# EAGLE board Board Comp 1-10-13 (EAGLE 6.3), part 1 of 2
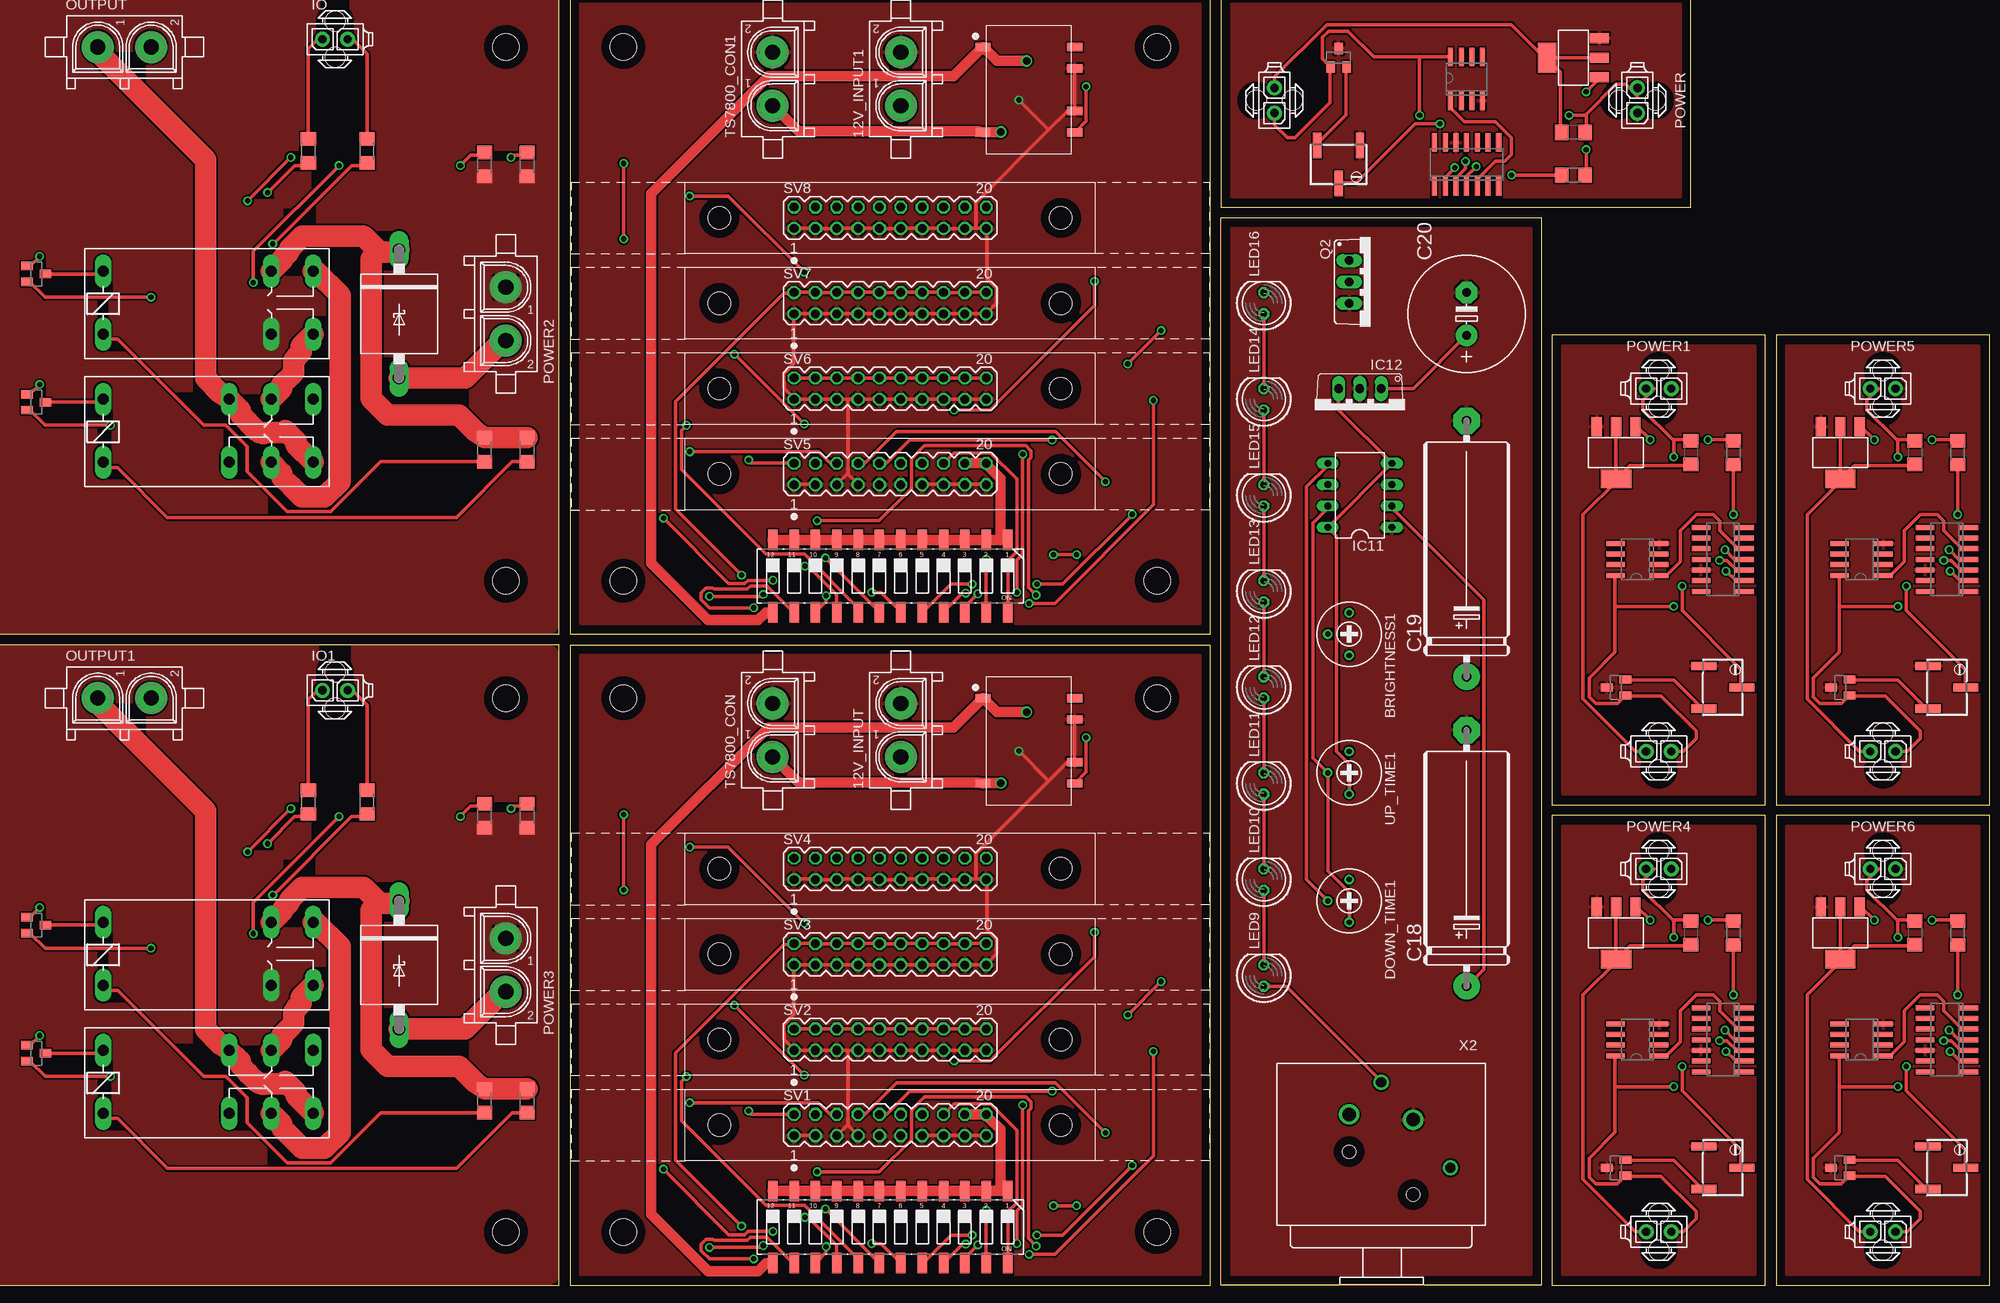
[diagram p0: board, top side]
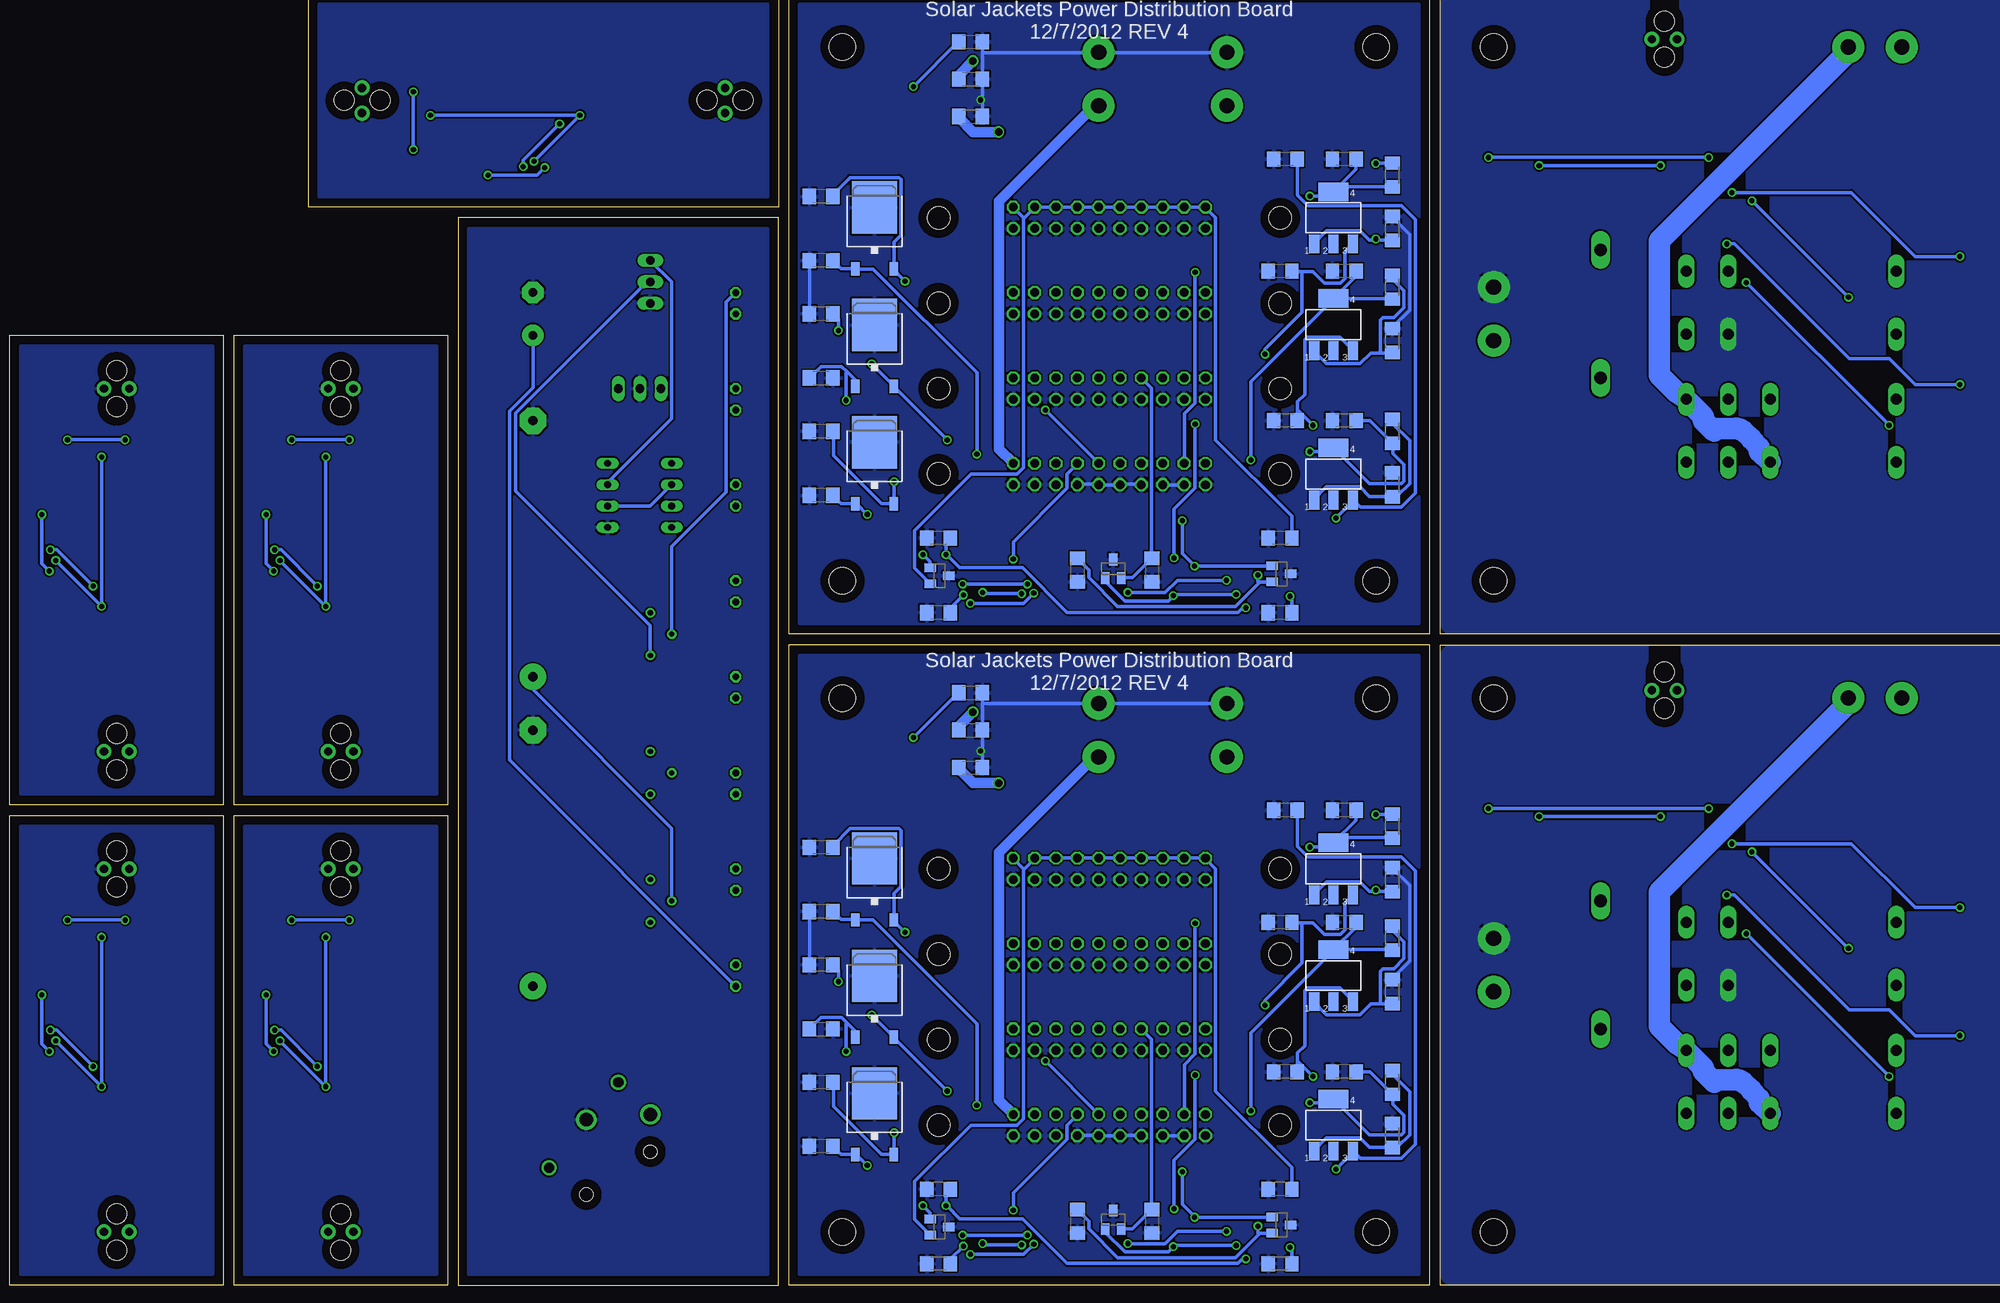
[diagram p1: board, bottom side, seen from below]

No outline drawn. Coordinates in mm, seen from the top.
Copper layers (1*16): Top 0.035mm / dielectric 1.5mm / Bottom 0.035mm
Design rules "default": minimum track width 10mil, minimum drill 24mil, track to track 8mil, track to pad 8mil, pad to pad 8mil, via to via 8mil, smd to smd 8mil, copper to edge 40mil, drill to drill 8mil, minimum pad ring 10mil, minimum via ring 8mil, stop-mask expansion 4mil, vias tented up to drill 0mil, thermal gap 10mil
Net classes: 1 power: width 1.27 mm, drill 0.889 mm
Holes 3.17 mm at 147.32,6.35 83.82,6.35 83.82,69.85 147.32,69.85 147.32,83.82 83.82,83.82 83.82,147.32 147.32,147.32 6.58,84 69.85,147.32 69.85,83.82 6.35,147.32 6.58,6.53 69.85,69.85 69.85,6.35 6.35,69.85
Milling: 40 lines

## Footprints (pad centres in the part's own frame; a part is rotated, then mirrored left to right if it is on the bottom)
SOT23 = smd 1 x 1.4: 1 -0.95,-1.1; 2 0.95,-1.1; 3 0,1.1
350759-4 = drill 1.8 pad 3.81: 1 -3.175,0; 2 3.175,0
C1206 = smd 1.6 x 1.8: 1 -1.4,0; 2 1.4,0
RTRIM3339P = drill 0.61: 1 -2.54,0; 2 0,-2.54; 3 2.54,0
E30-10 = drill 1.118 pad 3.15: + -15.24,0 | drill 1.118 pad 3.15 octagon: - 15.24,0
E5-13 = drill 1.016 pad 2.54: + -2.54,0 | drill 1.016 pad 2.54 octagon: - 2.54,0
P6T15 = drill 1.499 long: A 7.62,0; C -7.62,0
SO14 = smd 0.6 x 2.2: 1 -3.81,-2.6; 2 -2.54,-2.6; 3 -1.27,-2.6; 4 0,-2.6; 5 1.27,-2.6; 6 2.54,-2.6; 7 3.81,-2.6; 8 3.81,2.6; 9 2.54,2.6; 10 1.27,2.6; 11 0,2.6; 12 -1.27,2.6; 13 -2.54,2.6; 14 -3.81,2.6
SOT223 = smd 1.219 x 2.235: 1 -2.311,-3.099; 2 0,-3.099; 3 2.311,-3.099 | smd 3.6 x 2.2: 4 0,3.099
DIL08 = drill 0.813 long: 1 -3.81,-3.81; 2 -1.27,-3.81; 3 1.27,-3.81; 4 3.81,-3.81; 5 3.81,3.81; 6 1.27,3.81; 7 -1.27,3.81; 8 -3.81,3.81
TO220V = drill 1.016 long: 1 -2.54,-2.54; 2 0,-2.54; 3 2.54,-2.54
794681-2 = drill 1 pad 1.778: 1 0,-1.5; 2 0,1.5 | hole 2.4: 2.13,0; -2.17,0
G2R2 = drill 1.321 long: 1 -2.54,-3.683; 2 -2.54,3.81; O1 12.471,3.81; O2 12.471,-3.683; P1 17.45,3.81; P2 17.45,-3.683; S1 22.454,3.81; S2 22.454,-3.683
G2R2A = drill 1.321 long: 1 -2.54,-3.683; 2 -2.54,3.81; P1 17.45,3.81; P2 17.45,-3.683; S1 22.454,3.81; S2 22.454,-3.683
LED5MM = drill 0.813 octagon: A -1.27,0; K 1.27,0
350428-1 = drill 1.8 pad 3.81: 1 -3.175,0; 2 3.175,0
TO252 = smd 1 x 1.6: 1 -2.28,-4.8; 2 2.28,-4.8 | smd 5.4 x 6.2: 3 0,2.5
TO220BV = drill 1.016 long: D 0,-2.54; G -2.54,-2.54; S 2.54,-2.54
RTRIMTS63Y = smd 1 x 3: 1 -2.55,-2.25; 2 0,2.25; 3 2.55,-2.25
R1206 = smd 1.6 x 1.803: 1 -1.422,0; 2 1.422,0
CTS-219-12 = smd 1.13 x 2.44: 1 -13.97,-4.3; 2 -11.43,-4.3; 3 -8.89,-4.3; 4 -6.35,-4.3; 5 -3.81,-4.3; 6 -1.27,-4.3; 7 1.27,-4.3; 8 3.81,-4.3; 9 6.35,-4.3; 10 8.89,-4.3; 11 11.43,-4.3; 12 13.97,-4.3; 13 13.97,4.3; 14 11.43,4.3; 15 8.89,4.3; 16 6.35,4.3; 17 3.81,4.3; 18 1.27,4.3; 19 -1.27,4.3; 20 -3.81,4.3; 21 -6.35,4.3; 22 -8.89,4.3; 23 -11.43,4.3; 24 -13.97,4.3
MA10-2 = drill 1.016 octagon: 1 -11.43,-1.27; 2 -11.43,1.27; 3 -8.89,-1.27; 4 -8.89,1.27; 5 -6.35,-1.27; 6 -6.35,1.27; 7 -3.81,-1.27; 8 -3.81,1.27; 9 -1.27,-1.27; 10 -1.27,1.27; 11 1.27,-1.27; 12 1.27,1.27; 13 3.81,-1.27; 14 3.81,1.27; 15 6.35,-1.27; 16 6.35,1.27; 17 8.89,-1.27; 18 8.89,1.27; 19 11.43,-1.27; 20 11.43,1.27 | hole 2.692: -20.32,0; 20.32,0
SO-08 = smd 0.6 x 2.2: 1 -1.905,-2.6; 2 -0.635,-2.6; 3 0.635,-2.6; 4 1.905,-2.6; 5 1.905,2.6; 6 0.635,2.6; 7 -0.635,2.6; 8 -1.905,2.6
V7805 = smd 0.991 x 1.803: 1 0,0.902; 5 10.16,0.902; 6 10.16,11.798; 7 7.62,11.798; 9 2.54,11.798; 10 0,11.798
NC3FAH2 = drill 1.6: 1 -3.81,0.635; 2 3.81,0 | drill 1.2: 3 0,-3.815; G -8.25,6.355 | hole 1.6: -3.81,9.525; 3.81,4.445

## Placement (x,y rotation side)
3V1  MAX6103  [SOT23]  95.1,84.63 270 bottom
3V2  MAX6103  [SOT23]  115.11,85.24 0 bottom
3V3  MAX6103  [SOT23]  95.1,7.16 270 bottom
3V4  MAX6103  [SOT23]  115.11,7.77 0 bottom
3V5  MAX6103  [SOT23]  135.79,6.93 270 bottom
3V6  MAX6103  [SOT23]  135.79,84.4 270 bottom
12V_INPUT  350759-4  [350759-4]  116.84,66.04 90 top
12V_INPUT1  350759-4  [350759-4]  116.84,143.51 90 top
317CAP1  .33uF  [C1206]  94.61,133.99 180 bottom
317CAP2  1uF  [C1206]  87.63,102.87 180 bottom
317CAP3  .33uF  [C1206]  94.61,56.52 180 bottom
317CAP4  .33uF  [C1206]  95.25,120.65 180 bottom
317CAP5  1uF  [C1206]  87.63,133.99 180 bottom
317CAP6  .33uF  [C1206]  94.61,102.87 180 bottom
317CAP7  1uF  [C1206]  87.63,120.65 180 bottom
317CAP8  1uF  [C1206]  87.63,25.4 180 bottom
317CAP9  .33uF  [C1206]  95.25,43.18 180 bottom
317CAP10  1uF  [C1206]  87.63,56.52 180 bottom
317CAP11  .33uF  [C1206]  94.61,25.4 180 bottom
317CAP12  1uF  [C1206]  87.63,43.18 180 bottom
6103CAP1  1uF  [C1206]  135.89,80.01 180 bottom
6103CAP2  1uF  [C1206]  119.38,85.09 270 bottom
6103CAP3  1uF  [C1206]  95.25,80.01 180 bottom
6103CAP4  1uF  [C1206]  110.49,85.09 270 bottom
6103CAP5  1uF  [C1206]  135.89,88.9 180 bottom
6103CAP6  1uF  [C1206]  95.25,88.9 180 bottom
6103CAP7  1uF  [C1206]  135.89,2.54 180 bottom
6103CAP8  1uF  [C1206]  119.38,7.62 270 bottom
6103CAP9  1uF  [C1206]  95.25,2.54 180 bottom
6103CAP10  1uF  [C1206]  110.49,7.62 270 bottom
6103CAP11  1uF  [C1206]  135.89,11.43 180 bottom
6103CAP12  1uF  [C1206]  95.25,11.43 180 bottom
BRIGHTNESS1  10 k  [RTRIM3339P]  170.18,77.47 270 top
C1  1 uF  [C1206]  196.85,137.16 180 top
C2  1 uF  [C1206]  210.82,99.06 270 top
C3  1uF  [C1206]  149.86,44.45 180 bottom
C4  1uF  [C1206]  149.86,52.07 180 bottom
C5  1uF  [C1206]  149.86,30.48 0 bottom
C6  1uF  [C1206]  149.86,38.1 180 bottom
C7  1uF  [C1206]  149.86,24.13 180 bottom
C8  1uF  [C1206]  149.86,16.51 180 bottom
C9  1uF  [C1206]  149.86,121.92 180 bottom
C10  1uF  [C1206]  149.86,129.54 180 bottom
C11  1uF  [C1206]  149.86,107.95 0 bottom
C12  1uF  [C1206]  149.86,115.57 180 bottom
C13  1uF  [C1206]  149.86,101.6 180 bottom
C14  1uF  [C1206]  149.86,93.98 180 bottom
C15  1 uF  [C1206]  237.49,99.06 270 top
C16  1 uF  [C1206]  237.49,41.91 270 top
C18  1uF  [E30-10]  184.15,50.8 90 top
C19  1uF  [E30-10]  184.15,87.63 90 top
C20  1000uF  [E5-13]  184.15,115.57 90 top
C21  1 uF  [C1206]  210.82,41.91 270 top
D1  6A4  [P6T15]  57.15,38.1 270 top
D3  6A4  [P6T15]  57.15,115.57 270 top
DOWN_TIME1  10k  [RTRIM3339P]  170.18,45.72 270 top
IC1  LM339D  [SO14]  184.15,133.35 0 top
IC2  LM339D  [SO14]  214.63,86.36 90 top
IC3  LM317  [SOT223]  88.9,96.52 0 bottom
IC4  LM317  [SOT223]  88.9,19.05 0 bottom
IC5  LM317  [SOT223]  88.9,49.53 0 bottom
IC6  LM317  [SOT223]  88.9,36.83 0 bottom
IC7  LM317  [SOT223]  88.9,127 0 bottom
IC8  LM317  [SOT223]  88.9,114.3 0 bottom
IC9  LM339D  [SO14]  241.3,86.36 90 top
IC10  LM339D  [SO14]  241.3,29.21 90 top
IC11  ICM7555  [DIL08]  171.45,93.98 90 top
IC12  7805TV  [TO220V]  171.45,104.14 180 top
IC13  LM339D  [SO14]  214.63,29.21 90 top
IO  794681-2  [794681-2]  49.53,148.25 270 top
IO1  794681-2  [794681-2]  49.53,70.78 270 top
J1  794681-2  [794681-2]  207.01,63.5 90 top
J2  794681-2  [794681-2]  161.29,140.97 0 top
J3  794681-2  [794681-2]  207.01,6.35 90 top
J4  794681-2  [794681-2]  233.68,63.5 90 top
J5  794681-2  [794681-2]  233.68,6.35 90 top
K1  G2R2  [G2R2]  24.47,101.6 0 top
K2  G2R2A  [G2R2A]  24.47,116.84 0 top
K3  G2R2  [G2R2]  24.47,24.13 0 top
K4  G2R2A  [G2R2A]  24.47,39.37 0 top
LED9  [LED5MM]  160.02,36.83 90 top
LED10  [LED5MM]  160.02,48.26 90 top
LED11  [LED5MM]  160.02,59.69 90 top
LED12  [LED5MM]  160.02,71.12 90 top
LED13  [LED5MM]  160.02,82.55 90 top
LED14  [LED5MM]  160.02,105.41 90 top
LED15  [LED5MM]  160.02,93.98 90 top
LED16  [LED5MM]  160.02,116.84 90 top
OUTPUT  350428-1  [350428-1]  24.47,147.32 0 top
OUTPUT1  350428-1  [350428-1]  24.47,69.85 0 top
POWER  794681-2  [794681-2]  204.47,140.97 0 top
POWER1  794681-2  [794681-2]  207.01,106.68 90 top
POWER2  350428-1  [350428-1]  69.85,115.57 270 top
POWER3  350428-1  [350428-1]  69.85,38.1 270 top
POWER4  794681-2  [794681-2]  207.01,49.53 90 top
POWER5  794681-2  [794681-2]  233.68,106.68 90 top
POWER6  794681-2  [794681-2]  233.68,49.53 90 top
PWR_1  7805DT  [TO252]  143.51,48.26 0 bottom
PWR_2  7805DT  [TO252]  143.51,34.29 0 bottom
PWR_3  7805DT  [TO252]  143.51,20.32 0 bottom
PWR_4  7805DT  [TO252]  143.51,125.73 0 bottom
PWR_5  7805DT  [TO252]  143.51,111.76 0 bottom
PWR_6  7805DT  [TO252]  143.51,97.79 0 bottom
Q2  IRF512  [TO220BV]  172.72,119.38 270 top
R1  10k  [RTRIMTS63Y]  168.91,133.35 180 top
R2  10k  [RTRIMTS63Y]  214.63,71.12 270 top
R3  220  [R1206]  81.92,101.6 90 bottom
R4  361  [R1206]  81.92,95.25 90 bottom
R5  220  [R1206]  81.92,132.08 90 bottom
R6  361  [R1206]  81.92,125.73 90 bottom
R7  220  [R1206]  81.92,24.13 90 bottom
R8  361  [R1206]  81.92,17.78 90 bottom
R9  220  [R1206]  81.92,54.61 90 bottom
R10  361  [R1206]  81.92,48.26 90 bottom
R11  220  [R1206]  81.92,41.27 90 bottom
R12  361  [R1206]  81.92,34.92 90 bottom
R13  220  [R1206]  81.92,118.75 90 bottom
R14  361  [R1206]  81.92,112.39 90 bottom
R15  1k  [R1206]  72.39,99.4 90 top
R16  1k  [R1206]  67.31,99.4 90 top
R17  1k  [R1206]  53.34,134.96 90 top
R18  1k  [R1206]  46.35,134.96 90 top
R19  0  [R1206]  67.31,133.35 90 top
R20  0  [R1206]  72.39,133.35 90 top
R21  1k  [R1206]  72.39,21.93 90 top
R22  1k  [R1206]  67.31,21.93 90 top
R23  1k  [R1206]  53.34,57.49 90 top
R24  1k  [R1206]  46.35,57.49 90 top
R25  0  [R1206]  67.31,55.88 90 top
R26  0  [R1206]  72.39,55.88 90 top
R27  10k  [RTRIMTS63Y]  214.63,13.97 270 top
R28  10k  [RTRIMTS63Y]  241.3,71.12 270 top
R29  10k  [RTRIMTS63Y]  241.3,13.97 270 top
S1  219-12  [CTS-219-12]  115.57,6.91 180 top
S2  219-12  [CTS-219-12]  115.57,84.38 180 top
SV1  AMPLATCH-20  [MA10-2]  115.57,19.05 0 top
SV2  AMPLATCH-20  [MA10-2]  115.57,29.21 0 top
SV3  AMPLATCH-20  [MA10-2]  115.57,39.37 0 top
SV4  AMPLATCH-20  [MA10-2]  115.57,49.53 0 top
SV5  AMPLATCH-20  [MA10-2]  115.57,96.52 0 top
SV6  AMPLATCH-20  [MA10-2]  115.57,106.68 0 top
SV7  AMPLATCH-20  [MA10-2]  115.57,116.84 0 top
SV8  AMPLATCH-20  [MA10-2]  115.57,127 0 top
T1  PMV56XN  [SOT23]  13.97,105.07 270 top
T2  PMV56XN  [SOT23]  13.97,120.31 270 top
T3  PMV56XN  [SOT23]  13.97,27.6 270 top
T4  PMV56XN  [SOT23]  13.97,42.84 270 top
TS7800_CON  350759-4  [350759-4]  101.6,66.04 90 top
TS7800_CON1  350759-4  [350759-4]  101.6,143.51 90 top
U$1  100  [R1206]  196.85,132.08 0 top
U$2  MAX6103  [SOT23]  168.91,146.05 0 top
U$3  NDT3055  [SOT223]  196.85,146.05 90 top
U$4  LM35  [SO-08]  184.15,143.51 0 top
U$5  100  [R1206]  215.9,99.06 90 top
U$6  MAX6103  [SOT23]  201.93,71.12 90 top
U$7  NDT3055  [SOT223]  201.93,99.06 180 top
U$8  LM35  [SO-08]  204.47,86.36 90 top
U$9  V7805  [V7805]  125.73,69.85 270 top
U$10  V7805  [V7805]  125.73,147.32 270 top
U$11  100  [R1206]  215.9,41.91 90 top
U$12  MAX6103  [SOT23]  201.93,13.97 90 top
U$13  NDT3055  [SOT223]  201.93,41.91 180 top
U$14  LM35  [SO-08]  204.47,29.21 90 top
U$15  100  [R1206]  242.57,99.06 90 top
U$16  MAX6103  [SOT23]  228.6,71.12 90 top
U$17  NDT3055  [SOT223]  228.6,99.06 180 top
U$18  LM35  [SO-08]  231.14,86.36 90 top
U$19  100  [R1206]  242.57,41.91 90 top
U$20  MAX6103  [SOT23]  228.6,13.97 90 top
U$21  NDT3055  [SOT223]  228.6,41.91 180 top
U$22  LM35  [SO-08]  231.14,29.21 90 top
UP_TIME1  10k  [RTRIM3339P]  170.18,60.96 270 top
V7805_C1  1uF  [C1206]  132.08,147.96 0 bottom
V7805_C2  1uF  [C1206]  132.08,143.51 0 bottom
V7805_C3  1uF  [C1206]  132.08,139.06 0 bottom
V7805_C4  1uF  [C1206]  132.08,70.48 0 bottom
V7805_C5  1uF  [C1206]  132.08,66.04 0 bottom
V7805_C6  1uF  [C1206]  132.08,61.59 0 bottom
X2  NC3FAH2  [NC3FAH2]  173.99,20.32 180 top

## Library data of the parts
3V1-3V6 U$1 U$2 U$4-U$6 U$8 U$11 U$12 U$14-U$16 U$18-U$20 U$22 = SolarJacketsADC
12V_INPUT 12V_INPUT1 J1-J5 POWER POWER1 POWER4-POWER6 = con-amp
317CAP1-317CAP12 6103CAP1-6103CAP12 C1-C16 C18-C21 R3-R14 V7805_C1-V7805_C6 = rcl
BRIGHTNESS1 DOWN_TIME1 R1 R2 R27-R29 UP_TIME1 = resistor
D1 D3 = diode
IC1-IC10 IC12 IC13 PWR_1-PWR_6 = linear
IC11 = maxim; MF: MAXIM; MPN: ICM7555IPA+; OC_FARNELL: 9663762; OC_NEWARK: 68K4387
IO IO1 = con-amp; DIR: DIR; ON: ON
K1 K3 = relay; MF: OMRON COMPONENTS USA; MPN: G2R-2-DC6; OC_FARNELL: unknown; OC_NEWARK: 89C5317
K2 K4 = relay; MPN: G2R-2A-DC24; OC_FARNELL: 6985269; OC_NEWARK: 36M5257
LED9-LED16 = led
OUTPUT OUTPUT1 TS7800_CON TS7800_CON1 = con-amp; NEG: -; POS: +
POWER2 POWER3 = con-amp; NEG: -; POS: +; VOLTAGE: 12V
Q2 = transistor-power
R15-R18 R21-R24 = SolarJacketsADC; PART_NUM: CR1206-FX-1001GLF
R19 R20 R25 R26 = SolarJacketsADC; PART_NUM: CR1206-J/-000ELF
S1 S2 = switch-dil; OC_FARNELL: unknown; OC_NEWARK: unknown
SV1-SV8 = SolarJacketsADC; PART_NUM: 5499160-1
T1-T4 = SolarJacketsADC; PART_NUM: PMV56XN,215
U$3 U$7 U$13 U$17 U$21 = SolarJacketsADC; PART_NUM: NDT3055
U$9 U$10 = V7805
X2 = con-neutrik_ag; MPN: NC3FAH2; OC_FARNELL: unknown; OC_NEWARK: 27B4208

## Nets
3.3V1: 317CAP8.1 IC4.4 R7.1 SV1.6
3.3V1_EN: 317CAP3.1 IC4.3 S1.19
3.3V1_EN1: 317CAP1.1 IC3.3 S2.19
3.3V2: 317CAP10.1 IC5.4 R9.1 SV1.4
3.3V2_EN: 317CAP9.1 IC5.3 S1.18
3.3V2_EN1: 317CAP4.1 IC7.3 S2.18
3.3V3: 317CAP12.1 IC6.4 R11.1 SV1.2
3.3V3_EN: 317CAP11.1 IC6.3 S1.17
3.3V3_EN1: 317CAP6.1 IC8.3 S2.17
3.3V4: 317CAP7.1 IC8.4 R13.1 SV5.2
3.3V5: 317CAP2.1 IC3.4 R3.1 SV5.6
3.3V6: 317CAP5.1 IC7.4 R5.1 SV5.4
5V1: C4.1 PWR_1.2 SV1.12
5V1_EN: C3.1 PWR_1.1 S1.22
5V1_EN1: C9.1 PWR_4.1 S2.22
5V2: C6.1 PWR_2.2 SV1.10
5V2_EN: C5.1 PWR_2.1 S1.21
5V2_EN1: C11.1 PWR_5.1 S2.21
5V3: C7.1 PWR_3.2 SV1.8
5V3_EN: C8.1 PWR_3.1 S1.20
5V3_EN1: C14.1 PWR_6.1 S2.20
5V4: C13.1 PWR_6.2 SV5.8
5V5: C12.1 PWR_5.2 SV5.10
5V6: C10.1 PWR_4.2 SV5.12
5V7: IC11.4 IC11.8 IC12.3 UP_TIME1.3
12V: C1.1 IC1.3 J2.1 POWER.2 U$2.1 U$4.8
12V1: C2.1 IC2.3 J1.1 POWER1.2 U$6.1 U$8.8
12V1_EN: S1.24 SV1.16
12V1_EN1: S2.24 SV5.16
12V2 [power]: 12V_INPUT.1 S1.1 S1.2 S1.3 S1.4 S1.5 S1.6 S1.7 S1.8 S1.9 S1.10 S1.11 S1.12 SV1.18 SV1.20
12V2_EN: S1.23 SV1.14
12V2_EN1: S2.23 SV5.14
12V3 [power]: 12V_INPUT1.1 S2.1 S2.2 S2.3 S2.4 S2.5 S2.6 S2.7 S2.8 S2.9 S2.10 S2.11 S2.12 SV5.18 SV5.20
12V4 [power]: D3.C K2.P1 R15.2 R16.2
12V5 [power]: D1.C K4.P1 R21.2 R22.2
12V6: C21.1 IC13.3 J3.1 POWER4.2 U$12.1 U$14.8
12V7: C15.1 IC9.3 J4.1 POWER5.2 U$16.1 U$18.8
12V8: C16.1 IC10.3 J5.1 POWER6.2 U$20.1 U$22.8
12V_PRE [power]: D3.A POWER2.2
12V_PRE1 [power]: D1.A POWER3.2
24V1: C20.+ IC12.1 LED9.A X2.3
DIR: IO.2 R17.2
DIR1: IO1.2 R23.2
GND: IC1.12 POWER.1 R1.1 U$2.3 U$3.3 U$4.4
GND1: IC2.12 POWER1.1 R2.1 U$6.3 U$7.3 U$8.4
GND2: 3V3.3 3V4.3 3V5.3 12V_INPUT.2 317CAP3.2 317CAP8.2 317CAP9.2 317CAP10.2 317CAP11.2 317CAP12.2 6103CAP7.2 6103CAP8.2 6103CAP9.2 6103CAP10.2 6103CAP11.2 6103CAP12.2 C3.2 C4.2 C5.2 C6.2 C7.2 C8.2 PWR_1.3 PWR_2.3 PWR_3.3 R8.2 R10.2 R12.2 SV1.1 SV1.3 SV1.5 SV1.7 SV1.9 SV1.11 SV1.13 SV1.15 SV1.17 SV1.19 SV2.1 SV2.3 SV2.5 SV2.7 SV2.9 SV2.11 SV2.13 SV2.15 SV2.17 SV2.19 SV3.1 SV3.3 SV3.5 SV3.7 SV3.9 SV3.11 SV3.13 SV3.15 SV3.17 SV3.19 SV4.1 SV4.3 SV4.5 SV4.7 SV4.9 SV4.11 SV4.13 SV4.15 SV4.17 SV4.19 TS7800_CON.2 U$9.7 U$9.9 V7805_C4.2 V7805_C5.2 V7805_C6.2
GND3: 3V1.3 3V2.3 3V6.3 12V_INPUT1.2 317CAP1.2 317CAP2.2 317CAP4.2 317CAP5.2 317CAP6.2 317CAP7.2 6103CAP1.2 6103CAP2.2 6103CAP3.2 6103CAP4.2 6103CAP5.2 6103CAP6.2 C9.2 C10.2 C11.2 C12.2 C13.2 C14.2 PWR_4.3 PWR_5.3 PWR_6.3 R4.2 R6.2 R14.2 SV5.1 SV5.3 SV5.5 SV5.7 SV5.9 SV5.11 SV5.13 SV5.15 SV5.17 SV5.19 SV6.1 SV6.3 SV6.5 SV6.7 SV6.9 SV6.11 SV6.13 SV6.15 SV6.17 SV6.19 SV7.1 SV7.3 SV7.5 SV7.7 SV7.9 SV7.11 SV7.13 SV7.15 SV7.17 SV7.19 SV8.1 SV8.3 SV8.5 SV8.7 SV8.9 SV8.11 SV8.13 SV8.15 SV8.17 SV8.19 TS7800_CON1.2 U$10.7 U$10.9 V7805_C1.2 V7805_C2.2 V7805_C3.2
GND4: IC9.12 POWER5.1 R28.1 U$16.3 U$17.3 U$18.4
GND5: C18.- C19.- C20.- IC11.1 IC12.2 Q2.S X2.1
GND6 [power]: K2.P2 POWER2.1 R19.1 R20.1
GND7 [power]: K4.P2 POWER3.1 R25.1 R26.1
GND8: IC13.12 POWER4.1 R27.1 U$12.3 U$13.3 U$14.4
GND9: IC10.12 POWER6.1 R29.1 U$20.3 U$21.3 U$22.4
MOTOR+ [power]: K1.O2 K1.S1 OUTPUT.2
MOTOR+1 [power]: K3.O2 K3.S1 OUTPUT1.2
MOTOR- [power]: K1.O1 K1.S2 OUTPUT.1
MOTOR-1 [power]: K3.O1 K3.S2 OUTPUT1.1
N$1: IC1.2 U$1.1
N$2: U$1.2 U$3.1
N$3: IC1.4 R1.2
N$4: R1.3 U$2.2
N$5: C1.2 J2.2 U$3.2 U$3.4
N$6: IC2.2 U$5.1
N$7: IC2.4 R2.2
N$8: IC1.5 U$4.1
N$9: R2.3 U$6.2
N$10: U$5.2 U$7.1
N$11: C2.2 J1.2 U$7.2 U$7.4
N$12: IC2.5 U$8.1
N$13: IC4.1 R7.2 R8.1
N$14: IC5.1 R9.2 R10.1
N$15: IC6.1 R11.2 R12.1
N$16: U$9.6 V7805_C4.1
N$17: IC3.1 R3.2 R4.1
N$18: IC7.1 R5.2 R6.1
N$19: IC8.1 R13.2 R14.1
N$20: U$10.6 V7805_C1.1
N$21: IC9.2 U$15.1
N$22: IC9.4 R28.2
N$23: R28.3 U$16.2
N$24: U$15.2 U$17.1
N$25: C15.2 J4.2 U$17.2 U$17.4
N$26: IC9.5 U$18.1
N$27: IC10.2 U$19.1
N$28: IC10.4 R29.2
N$29: R29.3 U$20.2
N$30: U$19.2 U$21.1
N$31: C16.2 J5.2 U$21.2 U$21.4
N$32: IC10.5 U$22.1
N$34: C18.+ IC11.2 IC11.6
N$35: C19.+ DOWN_TIME1.2 IC11.5
N$36: DOWN_TIME1.3 IC11.7 UP_TIME1.2
N$37: LED9.K LED10.A
N$38: LED10.K LED11.A
N$39: LED11.K LED12.A
N$40: LED12.K LED13.A
N$41: LED13.K LED15.A
N$42: LED14.A LED15.K
N$43: LED14.K LED16.A
N$44: BRIGHTNESS1.2 LED16.K
N$45: BRIGHTNESS1.3 Q2.D
N$46: IC11.3 Q2.G
N$47 [power]: K1.P2 K2.S1
N$48 [power]: K1.P1 K2.S2
N$49: K1.1 R15.1
N$50: K2.1 R16.1
N$51: K1.2 T1.3
N$52: K2.2 T2.3
N$53: R18.1 T2.1
N$54: R17.1 T1.1
N$55: R19.2 T1.2
N$56: R20.2 T2.2
N$57 [power]: K3.P2 K4.S1
N$58 [power]: K3.P1 K4.S2
N$59: K3.1 R21.1
N$60: K4.1 R22.1
N$61: K3.2 T3.3
N$62: K4.2 T4.3
N$63: R24.1 T4.1
N$64: R23.1 T3.1
N$65: R25.2 T3.2
N$66: R26.2 T4.2
N$67: IC13.2 U$11.1
N$68: IC13.4 R27.2
N$69: R27.3 U$12.2
N$70: U$11.2 U$13.1
N$71: C21.2 J3.2 U$13.2 U$13.4
N$72: IC13.5 U$14.1
ON: IO.1 R18.2
ON1: IO1.1 R24.2
TS7800_+ [power]: TS7800_CON.1 U$9.5 V7805_C6.1
TS7800_+1 [power]: TS7800_CON1.1 U$10.5 V7805_C3.1
TS7800_EN [power]: S1.13 U$9.1 V7805_C5.1
TS7800_EN1 [power]: S2.13 U$10.1 V7805_C2.1
VREF1: 3V3.2 6103CAP8.1 SV3.2 SV3.4 SV3.6 SV3.8 SV3.10 SV3.12 SV3.14 SV3.16 SV3.18 SV3.20
VREF1_EN: 3V3.1 6103CAP7.1 S1.16
VREF1_EN1: 3V1.1 6103CAP1.1 S2.16
VREF2: 3V4.2 6103CAP10.1 SV2.2 SV2.4 SV2.6 SV2.8 SV2.10 SV2.12 SV2.14 SV2.16 SV2.18 SV2.20
VREF2_EN: 3V4.1 6103CAP9.1 S1.15
VREF2_EN1: 3V2.1 6103CAP3.1 S2.15
VREF3: 3V5.2 6103CAP12.1 SV4.2 SV4.4 SV4.6 SV4.8 SV4.10 SV4.12 SV4.14 SV4.16 SV4.18 SV4.20
VREF3_EN: 3V5.1 6103CAP11.1 S1.14
VREF3_EN1: 3V6.1 6103CAP5.1 S2.14
VREF4: 3V1.2 6103CAP2.1 SV7.2 SV7.4 SV7.6 SV7.8 SV7.10 SV7.12 SV7.14 SV7.16 SV7.18 SV7.20
VREF5: 3V2.2 6103CAP4.1 SV6.2 SV6.4 SV6.6 SV6.8 SV6.10 SV6.12 SV6.14 SV6.16 SV6.18 SV6.20
VREF6: 3V6.2 6103CAP6.1 SV8.2 SV8.4 SV8.6 SV8.8 SV8.10 SV8.12 SV8.14 SV8.16 SV8.18 SV8.20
